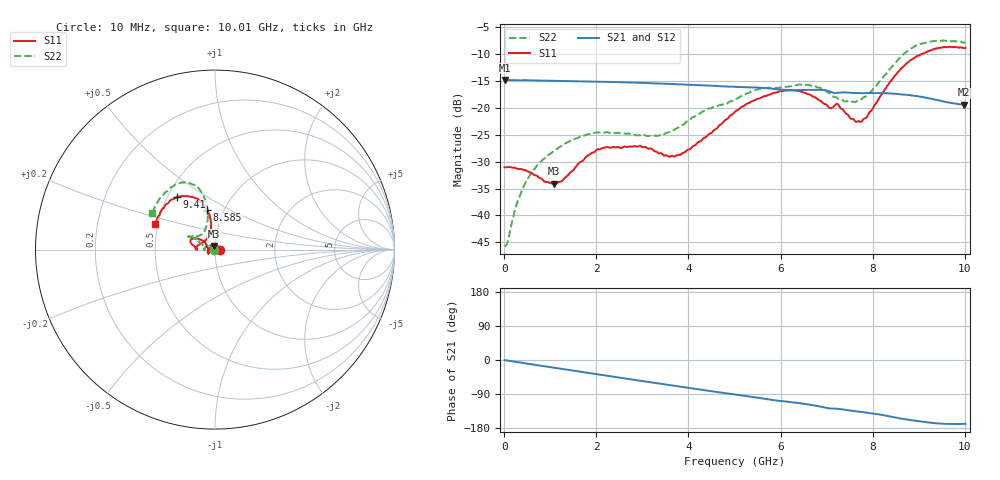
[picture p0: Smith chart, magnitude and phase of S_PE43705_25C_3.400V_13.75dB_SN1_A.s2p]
! Device ID: PE43705
! Serial: 1
! Insertion: A
! Impedance: 50 ohm
! Temp: 25C
! VDD: 3.400V
! Attenuation Step: 13.75dB
#  Hz  S  RI  R  50
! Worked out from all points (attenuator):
!   401 points, 10 MHz to 10.01 GHz, reference 50 ohm
!   highest |S21| = -14.78 dB at 10 MHz (marker M1); lowest = -19.4 dB at 9.985 GHz (marker M2)
!   lowest |S11| = -34.1 dB at 1.085 GHz (marker M3), VSWR 1.04, Z = 49.4 + j1.86 ohm
!   |S11| at or under -10 dB: start of sweep to 9.049 GHz
!   |S22| runs from -45.7 to -7.4 dB; largest |S21 - S12| = 0.0016
!   S11 on the Smith chart (normalised r, x): 10 MHz: 1.06, +0.00; 8.585 GHz: 0.83, +0.39; 9.41 GHz: 0.56, +0.38; 10.01 GHz: 0.48, +0.16
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1e7  0.0281 0.000239  0.1823 -0.000854  0.1826 -0.000689  -0.00516 0.000444
8.5e7  0.0281 0.00253  0.1818 -0.00544  0.1818 -0.00542  -0.00463 0.00351
2.85e8  0.0254 0.00956  0.1804 -0.0174  0.1804 -0.0173  -0.00618 0.0117
4.6e8  0.0215 0.0153  0.1791 -0.028  0.1791 -0.0276  -0.00918 0.0179
1.085e9  -0.00574 0.0189  0.1676 -0.0626  0.1677 -0.0626  -0.0319 0.0241
1.685e9  -0.0315 0.00472  0.1511 -0.0925  0.1512 -0.0924  -0.0527 0.0149
2.21e9  -0.0412 -0.0127  0.132 -0.1152  0.132 -0.1151  -0.0594 0.00351
2.96e9  -0.0386 -0.022  0.0986 -0.1403  0.0988 -0.1402  -0.0554 0.00352
3.36e9  -0.0341 -0.0164  0.0792 -0.1493  0.0793 -0.1491  -0.055 0.00711
3.86e9  -0.0376 0.00374  0.0539 -0.1567  0.054 -0.1566  -0.0661 0.021
5.01e9  -0.075 0.0539  -0.00288 -0.1574  -0.00249 -0.1574  -0.1061 0.0584
5.985e9  -0.1307 0.059  -0.0454 -0.1413  -0.0448 -0.1414  -0.1353 0.0749
6.685e9  -0.1262 0.0271  -0.0718 -0.1288  -0.0717 -0.1289  -0.1436 0.0722
7.36e9  -0.0925 0.026  -0.0912 -0.106  -0.0908 -0.106  -0.0874 0.0775
7.71e9  -0.0519 0.0545  -0.1 -0.0948  -0.0998 -0.095  -0.0606 0.1009
7.91e9  -0.0325 0.0822  -0.1049 -0.0889  -0.1047 -0.0897  -0.0494 0.1277
8.36e9  -0.0244 0.1691  -0.1169 -0.0711  -0.1166 -0.0719  -0.0434 0.2241
8.585e9  -0.0443 0.2199  -0.1203 -0.0588  -0.1197 -0.0597  -0.0591 0.2862
8.935e9  -0.0971 0.284  -0.1223 -0.0432  -0.1218 -0.0424  -0.1177 0.3613
9.41e9  -0.2116 0.2923  -0.1156 -0.0258  -0.1155 -0.0259  -0.2184 0.3642
9.985e9  -0.3275 0.1488  -0.1051 -0.0211  -0.1054 -0.0214  -0.3443 0.2129
1.001e10  -0.3349 0.1399  -0.1058 -0.0216  -0.1059 -0.0221  -0.3522 0.2022
